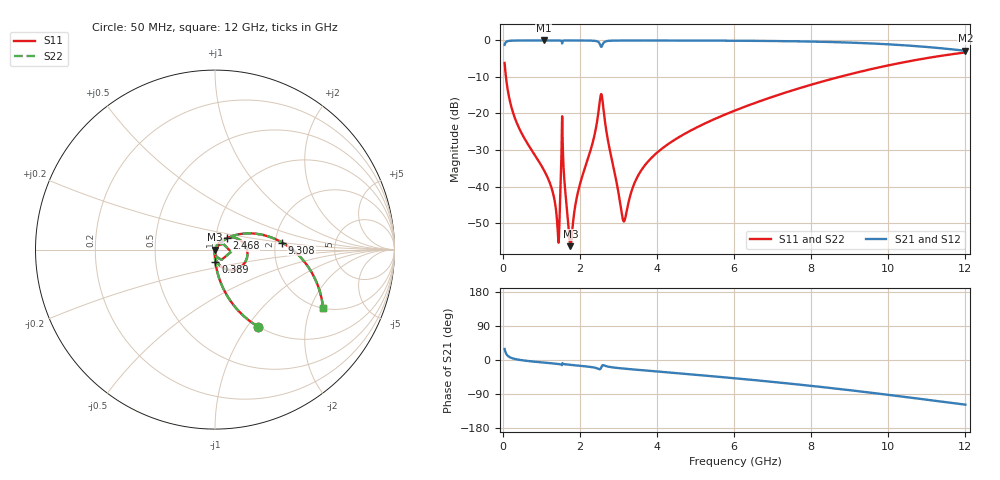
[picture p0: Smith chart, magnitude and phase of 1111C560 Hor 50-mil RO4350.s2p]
# GHz S MA R 50
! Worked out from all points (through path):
!   11951 points, 50 MHz to 12 GHz, reference 50 ohm
!   highest |S21| = -0.01 dB at 1.059 GHz (marker M1); lowest = -2.8 dB at 12 GHz (marker M2)
!   group delay of S21, straight-line fit = 27.5 ps
!   lowest |S11| = -56.3 dB at 1.757 GHz (marker M3), VSWR 1.00, Z = 50.1 - j0.0374 ohm
!   |S11| at or under -10 dB: 84.67 MHz to 8.729 GHz (8.644 GHz wide, 196 % of centre)
!   |S22| runs from -56.3 to -3.3 dB; largest |S21 - S12| = 0
!   S11 on the Smith chart (normalised r, x): 50 MHz: 0.99, -1.13; 389 MHz: 0.99, -0.14; 2.468 GHz: 1.13, +0.15; 9.308 GHz: 2.19, +0.20; 12 GHz: 2.01, -2.47
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0.05  0.492 -60.9  0.8703 29.1  0.8703 29.1  0.492 -60.9
0.197  0.1406 -83.2  0.9896 6.6  0.9896 6.6  0.1406 -83.2
0.389  0.0695 -88.3  0.9969 1.1  0.9969 1.1  0.0695 -88.3
1.059  0.01718 -93.3  0.9987 -6.8  0.9987 -6.8  0.01718 -93.3
1.29  0.008711 -90.9  0.9987 -8.9  0.9987 -8.9  0.008711 -90.9
1.428  0.002427 -61.1  0.9984 -10.3  0.9984 -10.3  0.002427 -61.1
1.466  0.002565 30.9  0.998 -10.8  0.998 -10.8  0.002565 30.9
1.528  0.03508 48.8  0.9828 -12.9  0.9828 -12.9  0.03508 48.8
1.566  0.02623 -85.9  0.9932 -10.0  0.9932 -10.0  0.02623 -85.9
1.702  0.003055 -72.7  0.9984 -12.3  0.9984 -12.3  0.003055 -72.7
1.757  0.001526 -14.1  0.9984 -12.8  0.9984 -12.8  0.001526 -14.1
2.042  0.01266 64.7  0.9977 -15.6  0.9977 -15.6  0.01266 64.7
2.468  0.0912 44.9  0.9616 -22.7  0.9616 -22.7  0.0912 44.9
2.582  0.1612 -43.0  0.8555 -14.3  0.8555 -14.3  0.1612 -43.0
3.14  0.00333 -19.8  0.9965 -22.7  0.9965 -22.7  0.00333 -19.8
3.493  0.01352 53.0  0.9971 -25.9  0.9971 -25.9  0.01352 53.0
4.034  0.03002 54.8  0.9969 -30.6  0.9969 -30.6  0.03002 54.8
6.025  0.1098 40.2  0.9906 -48.3  0.9906 -48.3  0.1098 40.2
8.017  0.249 20.7  0.9641 -68.4  0.9641 -68.4  0.249 20.7
9.308  0.377 5.9  0.9209 -83.3  0.9209 -83.3  0.377 5.9
10.009  0.4563 -2.7  0.884 -92.0  0.884 -92.0  0.4563 -2.7
12  0.6849 -28.4  0.7214 -117.9  0.7214 -117.9  0.6849 -28.4
